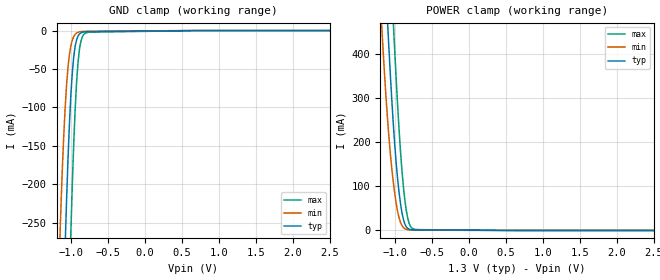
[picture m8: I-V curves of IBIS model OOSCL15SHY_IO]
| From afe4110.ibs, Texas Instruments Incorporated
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|   OOSCL15SHYIO model
[Model]   OOSCL15SHY_IO
Model_type   Input
Vinl =  0.39V |0.275V for 1.1V
Vinh =  0.91V |0.825V for 1.1V
|   typ   min   max
|   (nom)   (fast)   (weak)
C_comp   0.5391pF   0.4362pF   0.6541pF
[Model Spec]
Vinl   0.39V   0.275V   0.465V
Vinh   0.91V   0.825V   1.085V
[Voltage Range]   1.300V   1.100V   1.550V
[Temperature Range]   27.0   85.0   0.0
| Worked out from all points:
|   GND clamp passes 1 mA (typ) near -0.39 V on its own axis
|   POWER clamp passes 1 mA (typ) near -0.39 V on its own axis
[GND Clamp]
|   Voltage   I(typ)   I(min)   I(max)
-1.3V     -1.202A    -838mA     -1.561A
-1.163V   -581.7mA   -296.5mA   -908.2mA
-1.143V   -501.4mA   -237.8mA   -819mA
-1.084V   -284.2mA   -102.4mA   -561.9mA
-1.065V   -222.7mA   -71.75mA   -481mA
-1.045V   -168.3mA   -48.23mA   -403.4mA
-1.006V   -83.96mA   -19.62mA   -261.9mA
-966.8mV  -33.79mA   -7.538mA   -146.3mA
-927.6mV  -11.64mA   -3.145mA   -65.89mA
-868.8mV  -2.913mA   -1.325mA   -13.22mA
-790.5mV  -1.484mA   -907.8uA   -2.675mA
2.6V      0A         0A         0A
[POWER Clamp]
|   Voltage   I(typ)   I(min)   I(max)
-1.3V     1.192A     853.1mA    1.531A
-1.182V   754mA      470mA      1.065A
-1.104V   481.7mA    258.6mA    764.1mA
-1.084V   418.2mA    215.3mA    691mA
-1.026V   246.9mA    112.2mA    479.8mA
-1.006V   198.7mA    85.91mA    413.2mA
-947.2mV  88.52mA    29.83mA    233.1mA
-908mV    41.78mA    11.54mA    138.7mA
-868.8mV  15.23mA    4.189mA    71.05mA
-810.1mV  3.098mA    1.37mA     16.37mA
-731.7mV  1.407mA    864uA      2.585mA
2.6V      0A         0A         0A
